| stm32mp131_133_135 TFBGA289 9x9
[IBIS ver]   4.2
[File name]   stm32mp131_133_135_tfbga289.ibs
[File Rev]   3.4
[Date]   06-03-2024
[Source]   Data Created at STMicroelectronics
[Disclaimer]  This information is for modeling purpose only and is
   not guaranteed.
   The information is subject to change without notice.
[Copyright]   Copyright 2024 STMicroelectronics Inc.
|  You might uncomment [Merged Pins] sections if handeled by the simulation tool
[Component] stm32mp131_133_135_tfbga289
[Manufacturer] STMicroelectronics
[Package]
| variable   typ   min   max
R_pkg  0  NA  NA
L_pkg  0  NA  NA
C_pkg  0  NA  NA
[Pin]   signal_name   model_name
H11  BYPASS_REG1V8  nc
G16  DDR_A0  PDDRIO_PAD
L15  DDR_A1  PDDRIO_PAD
J15  DDR_A10  PDDRIO_PAD
L16  DDR_A11  PDDRIO_PAD
L14  DDR_A12  PDDRIO_PAD
E17  DDR_A13  PDDRIO_PAD
L17  DDR_A14  PDDRIO_PAD
K15  DDR_A15  PDDRIO_PAD
G13  DDR_A2  PDDRIO_PAD
G15  DDR_A3  PDDRIO_PAD
P15  DDR_A4  PDDRIO_PAD
F16  DDR_A5  PDDRIO_PAD
M15  DDR_A6  PDDRIO_PAD
F15  DDR_A7  PDDRIO_PAD
M16  DDR_A8  PDDRIO_PAD
F17  DDR_A9  PDDRIO_PAD
N17  DDR_ATO  nc
H15  DDR_BA0  PDDRIO_PAD
M17  DDR_BA1  PDDRIO_PAD
G14  DDR_BA2  PDDRIO_PAD
J17  DDR_CASN  PDDRIO_PAD
L13  DDR_CKE  PDDRIO_PAD
K17  DDR_CLKN  PDDRIO_PAD
K16  DDR_CLKP  PDDRIO_PAD
H16  DDR_CSN  PDDRIO_PAD
A16  DDR_DQ0  PDDRIO_PAD
B15  DDR_DQ1  PDDRIO_PAD
U16  DDR_DQ10  PDDRIO_PAD
R16  DDR_DQ11  PDDRIO_PAD
R15  DDR_DQ12  PDDRIO_PAD
T14  DDR_DQ13  PDDRIO_PAD
T15  DDR_DQ14  PDDRIO_PAD
U15  DDR_DQ15  PDDRIO_PAD
C14  DDR_DQ2  PDDRIO_PAD
C16  DDR_DQ3  PDDRIO_PAD
A15  DDR_DQ4  PDDRIO_PAD
C17  DDR_DQ5  PDDRIO_PAD
D17  DDR_DQ6  PDDRIO_PAD
D16  DDR_DQ7  PDDRIO_PAD
P17  DDR_DQ8  PDDRIO_PAD
R17  DDR_DQ9  PDDRIO_PAD
C15  DDR_DQM0  PDDRIO_PAD
R14  DDR_DQM1  PDDRIO_PAD
B16  DDR_DQS0N  PDIFF_PAD
B17  DDR_DQS0P  PDIFF_PAD
T17  DDR_DQS1N  PDIFF_PAD
T16  DDR_DQS1P  PDIFF_PAD
G17  DDR_ODT  PDDRIO_PAD
J14  DDR_RASN  PDDRIO_PAD
D15  DDR_RESETN  PDDRIO_PAD
J13  DDR_VREF  nc
H17  DDR_WEN  PDDRIO_PAD
P16  DDR_ZQ  nc
R10  NJTRST  io8_ft
K10  NRST  nc
J10  NRST_CORE  nc
L7  PA0  io8_ft
K8  PA1  io8_ft
J12  PA10  io8usb_id_otg20_ft
N5  PA11  io8_ft_i2c
F2  PA12  io8_ft_hslv
K7  PA13  io8_ft
R11  PA14  io8_ft
E7  PA15  io8_ft_hslv
R5  PA2  io8_ft
T7  PA3  io8_ft_hslv
N7  PA4  io8_ft
M7  PA5  io8_ft
R8  PA6  io8_ft_hslv
R6  PA7  io8_ft_hslv
J8  PA8  io8_ft_i2c_hslv
D2  PA9  io8_ft_hslv
M8  PB0  io8_ft
N8  PB1  io8_ft_hslv
G10  PB10  io8_ft_hslv
M6  PB11  io8_ft_hslv_et
A7  PB12  io8_ft_hslv
B10  PB13  io8_ft_i2c_hslv
A12  PB14  io8_ft_hslv
D11  PB15  io8_ft_hslv
K3  PB2  io8_ft_hslv
B11  PB3  io8_ft_hslv
E11  PB4  io8_ft_hslv
F9  PB5  io8_ft_hslv
G3  PB6  io8_ft_hslv
D5  PB7  io8_ft_i2c
G4  PB8  io8_ft_i2c
C10  PB9  io8_ft_i2c_hslv
T4  PC0  io8_ft_hslv
R7  PC1  io8_ft_hslv_et
F11  PC10  io8_ft_i2c_hslv
C12  PC11  io8_ft_i2c_hslv
B13  PC12  io8_ft_hslv
M3  PC13  io8_ft
M1  PC14  io8_ft
M2  PC15  io8_ft
U8  PC2  io8_ft_hslv_et
P7  PC3  io8_ft_hslv
K9  PC4  io8_ft
P8  PC5  io8_ft
A10  PC6  io8_ft_hslv
A9  PC7  io8_ft_hslv
C13  PC8  io8_ft_hslv
G12  PC9  io8_ft_hslv
E1  PD0  io8_ft
C2  PD1  io8_ft_i2c_hslv
D3  PD10  io8_ft_hslv
G1  PD11  io8_ft_hslv
D7  PD12  io8_ft_i2c
N1  PD13  io8_ft_hslv
F7  PD14  io8_ft_i2c_hslv
A5  PD15  io8_ft_hslv
G11  PD2  io8_ft_hslv
G6  PD3  io8_ft_i2c
A2  PD4  io8_ft_hslv
B4  PD5  io8_ft_hslv
G9  PD6  io8_ft
R3  PD7  io8_ft_i2c_hslv
B2  PD8  io8_ft
B5  PD9  io8_ft_hslv
U7  PDR_ON  nc
B3  PE0  io8_ft_hslv
C3  PE1  io8_ft_hslv
C7  PE10  io8_ft
E4  PE11  io8_ft_hslv_et
B1  PE12  io8_ft_hslv
C1  PE13  io8_ft_i2c_hslv
E2  PE14  io8_ft_hslv
A6  PE15  io8_ft_i2c_hslv
T1  PE2  io8_ft_i2c_hslv
B12  PE3  io8_ft_hslv
K1  PE4  io8_ft_hslv
L9  PE5  io8_ft_hslv_et
R2  PE6  io8_ft_hslv_et
C4  PE7  io8_ft_hslv
F8  PE8  io8_ft_i2c
A3  PE9  io8_ft_hslv
A11  PF0  io8_ft_hslv
A8  PF1  io8_ft_i2c_hslv
K2  PF10  io8_ft_hslv
L8  PF11  io8_ft
J9  PF12  io8_ft_hslv_et
T3  PF13  io8_ft
U4  PF14  io8_ft
L10  PF15  io8_ft
B7  PF2  io8_ft_i2c_hslv
B9  PF3  io8_ft_i2c_hslv
P3  PF4  io8_ft_hslv
D1  PF5  io8_ft_hslv
L1  PF6  io8_ft_hslv_et
J7  PF7  io8_ft_hslv_et
H3  PF8  io8_ft_hslv
H9  PF9  io8_ft_hslv
A4  PG0  io8_ft_hslv
P4  PG1  io8_ft_hslv_et
H2  PG10  io8_ft_hslv
R1  PG11  io8_ft_hslv_et
L6  PG12  io8_ft
R9  PG13  io8_ft_hslv_et
T8  PG14  io8_ft_hslv_et
G8  PG15  io8_ft_hslv
U3  PG2  io8_ft
U2  PG3  io8_ft_et_i2c_hslv
C9  PG4  io8_ft_hslv
H1  PG5  io8_ft_hslv
H10  PG6  io8_ft_hslv
C8  PG7  io8_ft_hslv
J3  PG8  io8_ft_hslv
G5  PG9  io8_ft_i2c
P1  PH0  io8_ft
P2  PH1  io8_ft
C11  PH10  io8_ft_hslv
H7  PH11  io8_ft_i2c_hslv
G7  PH12  io8_ft_i2c_hslv
E9  PH13  io8_ft_i2c_hslv
B6  PH14  io8_ft_i2c_hslv
G2  PH2  io8_ft_hslv
T2  PH3  io8_ft_i2c_hslv
T13  PH4  io8_ft
L12  PH5  io8_ft
J6  PH6  io8_ft_i2c_hslv
L3  PH7  io8_ft_i2c_hslv
F1  PH8  io8_ft_i2c_hslv
D9  PH9  io8_ft_hslv
N3  PI0  io8_ft
N4  PI1  io8_ft
J4  PI2  io8_ft
H8  PI3  io8_ft
P11  PI4  io8_ft
N11  PI5  io8_ft
M11  PI6  io8_ft
U13  PI7  io8usb_vbus_otg20_ft
R4  PWR_CPU_ON  io8_ft
U14  PWR_LP  io8_ft
R13  PWR_ON  io8_ft
U12  USB_DM1  nc
U9  USB_DM2  nc
T12  USB_DP1  nc
T9  USB_DP2  nc
M10  USB_RREF  nc
J5  VBAT  power
L4  VDD_ANA  power
C6  VDD  power
F6  VDD_CORE  power
F10  VDD_CORE  power
F12  VDD_CORE  power
H6  VDD_CORE  power
H12  VDD_CORE  power
K12  VDD_CORE  power
M12  VDD_CORE  power
K6  VDD_CORE  power
M9  VDD_CORE  power
D4  VDD_CPU  power
D6  VDD_CPU  power
D8  VDD_CPU  power
E5  VDD_CPU  power
F4  VDD_CPU  power
H4  VDD_CPU  power
D10  VDD  power
D12  VDD  power
D14  VDD_DDR  power
E13  VDD_DDR  power
E15  VDD_DDR  power
F14  VDD_DDR  power
H14  VDD_DDR  power
K14  VDD_DDR  power
M14  VDD_DDR  power
N13  VDD_DDR  power
N15  VDD_DDR  power
P14  VDD_DDR  power
F3  VDD  power
K4  VDD  power
M4  VDD  power
P12  VDD  power
P6  VDD  power
P9  VDD  power
P10  VDD  power
J1  VDD_PLL  power
L11  VDD_PLL2  power
U11  VDD3V3_USBHS  power
U5  VDDA  power
U10  VDDA1V1_REG  power
J11  VDDA1V8_REG  power
A14  VDDSDMMC1  power
A13  VDDSDMMC2  power
T6  VREFN  gnd
U6  VREFP  power
A1  VSS  gnd
A17  VSS  gnd
B8  VSS  gnd
B14  VSS  gnd
C5  VSS  gnd
D13  VSS  gnd
E3  VSS  gnd
E6  VSS  gnd
E8  VSS  gnd
E10  VSS  gnd
E12  VSS  gnd
E14  VSS  gnd
E16  VSS  gnd
F5  VSS  gnd
F13  VSS  gnd
H5  VSS  gnd
H13  VSS  gnd
J16  VSS  gnd
K5  VSS  gnd
K13  VSS  gnd
M5  VSS  gnd
M13  VSS  gnd
N6  VSS  gnd
N9  VSS  gnd
N10  VSS  gnd
N12  VSS  gnd
N14  VSS  gnd
N16  VSS  gnd
P5  VSS  gnd
P13  VSS  gnd
U17  VSS  gnd
L5  VSS_ANA  gnd
L2  VSS  gnd
N2  VSS  gnd
U1  VSS  gnd
J2  VSS_PLL  gnd
K11  VSS_PLL2  gnd
R12  VSS  gnd
T10  VSS  gnd
T11  VSS_USBHS  gnd
T5  VSSA  gnd
[Package Model]   501-bga-9x9-289-210615
[Pin Mapping]   pulldown_ref   pullup_ref   | Comment
H11  nc  nc  | Depending on IO usage
| H11  nc  nc  | Depending on IO usage
G16  gnd  vddddr
L15  gnd  vddddr
J15  gnd  vddddr
L16  gnd  vddddr
L14  gnd  vddddr
E17  gnd  vddddr
L17  gnd  vddddr
K15  gnd  vddddr
G13  gnd  vddddr
G15  gnd  vddddr
P15  gnd  vddddr
F16  gnd  vddddr
M15  gnd  vddddr
F15  gnd  vddddr
M16  gnd  vddddr
F17  gnd  vddddr
N17  nc  nc
H15  gnd  vddddr
M17  gnd  vddddr
G14  gnd  vddddr
J17  gnd  vddddr
L13  gnd  vddddr
K17  gnd  vddddr
K16  gnd  vddddr
H16  gnd  vddddr
A16  gnd  vddddr
B15  gnd  vddddr
U16  gnd  vddddr
R16  gnd  vddddr
R15  gnd  vddddr
T14  gnd  vddddr
T15  gnd  vddddr
U15  gnd  vddddr
C14  gnd  vddddr
C16  gnd  vddddr
A15  gnd  vddddr
C17  gnd  vddddr
D17  gnd  vddddr
D16  gnd  vddddr
P17  gnd  vddddr
R17  gnd  vddddr
C15  gnd  vddddr
R14  gnd  vddddr
B16  gnd  vddddr
B17  gnd  vddddr
T17  gnd  vddddr
T16  gnd  vddddr
G17  gnd  vddddr
J14  gnd  vddddr
D15  gnd  vddddr
J13  nc  nc
H17  gnd  vddddr
P16  nc  nc
R10  gnd  vddio
K10  nc  nc
J10  nc  nc
L7  gnd  vddio
K8  gnd  vddio
J12  gnd  vddio
N5  gnd  vddio
F2  gnd  vddio
K7  gnd  vddio
R11  gnd  vddio
E7  gnd  vddio
R5  gnd  vddio
T7  gnd  vddio
N7  gnd  vddio
M7  gnd  vddio
R8  gnd  vddio
R6  gnd  vddio
J8  gnd  vddio
D2  gnd  vddio
M8  gnd  vddio
N8  gnd  vddio
G10  gnd  vddio
M6  gnd  vddio
A7  gnd  vddio
B10  gnd  vddio
A12  gnd  vdds2  | Depending on IO usage
| A12  gnd  vddio  | Depending on IO usage
D11  gnd  vdds2  | Depending on IO usage
| D11  gnd  vddio  | Depending on IO usage
K3  gnd  vddio
B11  gnd  vdds2  | Depending on IO usage
| B11  gnd  vddio  | Depending on IO usage
E11  gnd  vdds2  | Depending on IO usage
| E11  gnd  vddio  | Depending on IO usage
F9  gnd  vddio
G3  gnd  vddio
D5  gnd  vddio
G4  gnd  vddio
C10  gnd  vddio
T4  gnd  vddio
R7  gnd  vddio
F11  gnd  vdds1  | Depending on IO usage
| F11  gnd  vddio  | Depending on IO usage
C12  gnd  vdds1  | Depending on IO usage
| C12  gnd  vddio  | Depending on IO usage
B13  gnd  vdds1  | Depending on IO usage
| B13  gnd  vddio  | Depending on IO usage
M3  gnd  vddio  | Depending on IO usage
| M3  gnd  vbat  | Depending on IO usage
M1  gnd  vddio  | Depending on IO usage
| M1  gnd  vbat  | Depending on IO usage
M2  gnd  vddio  | Depending on IO usage
| M2  gnd  vbat  | Depending on IO usage
U8  gnd  vddio
P7  gnd  vddio
K9  gnd  vddio
P8  gnd  vddio
A10  gnd  vddio
A9  gnd  vddio
C13  gnd  vdds1  | Depending on IO usage
| C13  gnd  vddio  | Depending on IO usage
G12  gnd  vdds1  | Depending on IO usage
| G12  gnd  vddio  | Depending on IO usage
E1  gnd  vddio
C2  gnd  vddio
D3  gnd  vddio
G1  gnd  vddio
D7  gnd  vddio
N1  gnd  vddio
F7  gnd  vddio
A5  gnd  vddio
G11  gnd  vdds1  | Depending on IO usage
| G11  gnd  vddio  | Depending on IO usage
G6  gnd  vddio
A2  gnd  vddio
B4  gnd  vddio
G9  gnd  vddio
R3  gnd  vddio
B2  gnd  vddio
B5  gnd  vddio
U7  nc  nc
B3  gnd  vddio
C3  gnd  vddio
C7  gnd  vddio
E4  gnd  vddio
B1  gnd  vddio
C1  gnd  vddio
E2  gnd  vddio
A6  gnd  vddio
T1  gnd  vddio
B12  gnd  vdds2  | Depending on IO usage
| B12  gnd  vddio  | Depending on IO usage
K1  gnd  vddio
L9  gnd  vddio
R2  gnd  vddio
C4  gnd  vddio
F8  gnd  vddio
A3  gnd  vddio
A11  gnd  vddio
A8  gnd  vddio
K2  gnd  vddio
L8  gnd  vddio
J9  gnd  vddio
T3  gnd  vddio
U4  gnd  vddio
L10  gnd  vddio
B7  gnd  vddio
B9  gnd  vddio
P3  gnd  vddio
D1  gnd  vddio
L1  gnd  vddio
J7  gnd  vddio
H3  gnd  vddio
H9  gnd  vddio
A4  gnd  vddio
P4  gnd  vddio
H2  gnd  vddio
R1  gnd  vddio
L6  gnd  vddio
R9  gnd  vddio
T8  gnd  vddio
G8  gnd  vddio
U3  gnd  vddio
U2  gnd  vddio
C9  gnd  vddio
H1  gnd  vddio
H10  gnd  vdds2  | Depending on IO usage
| H10  gnd  vddio  | Depending on IO usage
C8  gnd  vddio
J3  gnd  vddio
G5  gnd  vddio
P1  gnd  vddio
P2  gnd  vddio
C11  gnd  vddio
H7  gnd  vddio
G7  gnd  vddio
E9  gnd  vddio
B6  gnd  vddio
G2  gnd  vddio
T2  gnd  vddio
T13  gnd  vddio
L12  gnd  vddio
J6  gnd  vddio
L3  gnd  vddio
F1  gnd  vddio
D9  gnd  vddio
N3  gnd  vddio
N4  gnd  vddio  | Depending on IO usage
| N4  gnd  vbat  | Depending on IO usage
J4  gnd  vddio  | Depending on IO usage
| J4  gnd  vbat  | Depending on IO usage
H8  gnd  vddio  | Depending on IO usage
| H8  gnd  vbat  | Depending on IO usage
P11  gnd  vddio
N11  gnd  vddio
M11  gnd  vddio
U13  gnd  vddio
R4  gnd  vddio
U14  gnd  vddio
R13  gnd  vddio
U12  nc  nc  | Depending on IO usage
| U12  nc  nc  | Depending on IO usage
U9  nc  nc  | Depending on IO usage
| U9  nc  nc  | Depending on IO usage
T12  nc  nc  | Depending on IO usage
| T12  nc  nc  | Depending on IO usage
T9  nc  nc  | Depending on IO usage
| T9  nc  nc  | Depending on IO usage
M10  nc  nc  | Depending on IO usage
| M10  nc  nc  | Depending on IO usage
J5  nc  vbat
L4  nc  vddana
C6  nc  vddio
F6  nc  vddio  | Depending on IO usage
| F6  nc  vbat  | Depending on IO usage
F10  nc  vddio  | Depending on IO usage
| F10  nc  vbat  | Depending on IO usage
F12  nc  vddio  | Depending on IO usage
| F12  nc  vbat  | Depending on IO usage
H6  nc  vddio  | Depending on IO usage
| H6  nc  vbat  | Depending on IO usage
H12  nc  vddio  | Depending on IO usage
| H12  nc  vbat  | Depending on IO usage
K12  nc  vddio  | Depending on IO usage
| K12  nc  vbat  | Depending on IO usage
M12  nc  vddio  | Depending on IO usage
| M12  nc  vbat  | Depending on IO usage
K6  nc  vddio  | Depending on IO usage
| K6  nc  vbat  | Depending on IO usage
M9  nc  vddio  | Depending on IO usage
| M9  nc  vbat  | Depending on IO usage
D4  nc  vddcpu
D6  nc  vddcpu
D8  nc  vddcpu
E5  nc  vddcpu
F4  nc  vddcpu
H4  nc  vddcpu
D10  nc  vddio
D12  nc  vddio
D14  nc  vddddr
E13  nc  vddddr
E15  nc  vddddr
F14  nc  vddddr
H14  nc  vddddr
K14  nc  vddddr
M14  nc  vddddr
N13  nc  vddddr
N15  nc  vddddr
P14  nc  vddddr
F3  nc  vddio
K4  nc  vddio
M4  nc  vddio
P12  nc  vddio
P6  nc  vddio
P9  nc  vddio
P10  nc  vddio
J1  nc  vddpll
L11  nc  vddpll2
U11  nc  vdd3v3usbhs
U5  nc  vdda
U10  nc  vdda1v1
J11  nc  vdda1v8
A14  nc  vdds1
A13  nc  vdds2
T6  gnd  nc
U6  nc  vddio
A1  gnd  nc
A17  gnd  nc
B8  gnd  nc
B14  gnd  nc
C5  gnd  nc
D13  gnd  nc
E3  gnd  nc
E6  gnd  nc
E8  gnd  nc
E10  gnd  nc
E12  gnd  nc
E14  gnd  nc
E16  gnd  nc
F5  gnd  nc
F13  gnd  nc
H5  gnd  nc
H13  gnd  nc
J16  gnd  nc
K5  gnd  nc
K13  gnd  nc
M5  gnd  nc
M13  gnd  nc
N6  gnd  nc
N9  gnd  nc
N10  gnd  nc
N12  gnd  nc
N14  gnd  nc
N16  gnd  nc
P5  gnd  nc
P13  gnd  nc
U17  gnd  nc
L5  gnd  nc
L2  gnd  nc
N2  gnd  nc
U1  gnd  nc
J2  gnd  nc
K11  gnd  nc
R12  gnd  nc
T10  gnd  nc
T11  gnd  nc
T5  gnd  nc
[Diff_pin]   inv_pin   vdiff   tdelay_typ   tdelay_min   tdelay_max
   K16   K17   0.320V   0ns   NA   NA   |CK
   B17   B16   0.320V   0ns   NA   NA   |DQS0
   T16   T17   0.320V   0ns   NA   NA   |DQS1
[Model Selector] PDIFF_PAD
MSD_D3RF2_18   DDR2 MSD_D3R_PDIFF Z0=18-Ohm
MSD_D3RF2_40   DDR2 MSD_D3R_PDIFF Z0=40-Ohm
MSD_D3RF2_48   DDR2 MSD_D3R_PDIFF Z0=48-Ohm
MSD_D3RF2_ODT150   DDR2 MSD_D3R_PDIFF cell 150-Ohm ODT Receiver
MSD_D3RF2_ODT50   DDR2 MSD_D3R_PDIFF cell 50-Ohm ODT Receiver
MSD_D3RF2_ODT75   DDR2 MSD_D3R_PDIFF cell 75-Ohm ODT Receiver
MSD_D3RF2_ODTOFF   DDR2 MSD_D3R_PDIFF cell ODT off Receiver
MSD_D3RF3_34   DDR3 MSD_D3R_PDIFF cell  Z0=34-Ohm
MSD_D3RF3_40   DDR3 MSD_D3R_PDIFF cell  Z0=40-Ohm
MSD_D3RF3_48   DDR3 MSD_D3R_PDIFF cell  Z0=48-Ohm
MSD_D3RF3L_34   DDR3L MSD_D3R_PDIFF cell  Z0=34-Ohm
MSD_D3RF3L_40   DDR3L MSD_D3R_PDIFF cell  Z0=40-Ohm
MSD_D3RF3L_48   DDR3L MSD_D3R_PDIFF cell  Z0=48-Ohm
MSD_D3RF3L_ODT120   DDR3L MSD_D3R_PDIFF cell 120-Ohm ODT Receiver
MSD_D3RF3L_ODT40   DDR3L MSD_D3R_PDIFF cell 40-Ohm ODT Receiver
MSD_D3RF3L_ODT60   DDR3L MSD_D3R_PDIFF cell 60-Ohm ODT Receiver
MSD_D3RF3L_ODTOFF   DDR3L MSD_D3R_PDIFF cell ODT off Receiver
MSD_D3RF3_ODT120   DDR3 MSD_D3R_PDIFF cell 120-Ohm ODT Receiver
MSD_D3RF3_ODT40   DDR3 MSD_D3R_PDIFF cell 40-Ohm ODT Receiver
MSD_D3RF3_ODT60   DDR3 MSD_D3R_PDIFF cell 60-Ohm ODT Receiver
MSD_D3RF3_ODTOFF   DDR3 MSD_D3R_PDIFF cell ODT off Receiver
MSD_D3RFL2_34   LPDDR2 MSD_D3R_PDIFF cell  Z0=34-Ohm
MSD_D3RFL2_40   LPDDR2 MSD_D3R_PDIFF cell  Z0=40-Ohm
MSD_D3RFL2_48   LPDDR2 MSD_D3R_PDIFF cell  Z0=48-Ohm
MSD_D3RFL2_60   LPDDR2 MSD_D3R_PDIFF cell  Z0=60-Ohm
MSD_D3RFL2_80   LPDDR2 MSD_D3R_PDIFF cell  Z0=80-Ohm
MSD_D3RFL2_ODTOFF   LPDDR2 MSD_D3R_PDIFF cell ODT off Receiver
MSD_D3RFL_48   LPDDR MSD_D3R_PDIFF cell  Z0=48-Ohm
MSD_D3RFL_ODTOFF   LPDDR MSD_D3R_PDIFF cell ODT off Receiver
MSD_D3RF2_18_OPEN   DDR2 MSD_D3R_PDIFF_PDQSR Z0=18-Ohm
MSD_D3RF2_40_OPEN   DDR2 MSD_D3R_PDIFF_PDQSR Z0=40-Ohm
MSD_D3RF2_48_OPEN   DDR2 MSD_D3R_PDIFF_PDQSR Z0=48-Ohm
MSD_D3RF2_18_PD344   DDR2 MSD_D3R_PDIFF_PDQSR Z0=18-Ohm
MSD_D3RF2_40_PD344   DDR2 MSD_D3R_PDIFF_PDQSR Z0=40-Ohm
MSD_D3RF2_48_PD344   DDR2 MSD_D3R_PDIFF_PDQSR Z0=48-Ohm
MSD_D3RF2_18_PD393   DDR2 MSD_D3R_PDIFF_PDQSR Z0=18-Ohm
MSD_D3RF2_40_PD393   DDR2 MSD_D3R_PDIFF_PDQSR Z0=40-Ohm
MSD_D3RF2_48_PD393   DDR2 MSD_D3R_PDIFF_PDQSR Z0=48-Ohm
MSD_D3RF2_18_PD458   DDR2 MSD_D3R_PDIFF_PDQSR Z0=18-Ohm
MSD_D3RF2_40_PD458   DDR2 MSD_D3R_PDIFF_PDQSR Z0=40-Ohm
MSD_D3RF2_48_PD458   DDR2 MSD_D3R_PDIFF_PDQSR Z0=48-Ohm
MSD_D3RF2_18_PD500   DDR2 MSD_D3R_PDIFF_PDQSR Z0=18-Ohm
MSD_D3RF2_40_PD500   DDR2 MSD_D3R_PDIFF_PDQSR Z0=40-Ohm
MSD_D3RF2_48_PD500   DDR2 MSD_D3R_PDIFF_PDQSR Z0=48-Ohm
MSD_D3RF2_18_PD550   DDR2 MSD_D3R_PDIFF_PDQSR Z0=18-Ohm
MSD_D3RF2_40_PD550   DDR2 MSD_D3R_PDIFF_PDQSR Z0=40-Ohm
MSD_D3RF2_48_PD550   DDR2 MSD_D3R_PDIFF_PDQSR Z0=48-Ohm
MSD_D3RF2_18_PD611   DDR2 MSD_D3R_PDIFF_PDQSR Z0=18-Ohm
MSD_D3RF2_40_PD611   DDR2 MSD_D3R_PDIFF_PDQSR Z0=40-Ohm
MSD_D3RF2_48_PD611   DDR2 MSD_D3R_PDIFF_PDQSR Z0=48-Ohm
MSD_D3RF2_18_PD688   DDR2 MSD_D3R_PDIFF_PDQSR Z0=18-Ohm
MSD_D3RF2_40_PD688   DDR2 MSD_D3R_PDIFF_PDQSR Z0=40-Ohm
MSD_D3RF2_48_PD688   DDR2 MSD_D3R_PDIFF_PDQSR Z0=48-Ohm
MSD_D3RF2_18_PU344   DDR2 MSD_D3R_PDIFF_PDQSR Z0=18-Ohm
MSD_D3RF2_40_PU344   DDR2 MSD_D3R_PDIFF_PDQSR Z0=40-Ohm
MSD_D3RF2_48_PU344   DDR2 MSD_D3R_PDIFF_PDQSR Z0=48-Ohm
MSD_D3RF2_18_PU393   DDR2 MSD_D3R_PDIFF_PDQSR Z0=18-Ohm
MSD_D3RF2_40_PU393   DDR2 MSD_D3R_PDIFF_PDQSR Z0=40-Ohm
MSD_D3RF2_48_PU393   DDR2 MSD_D3R_PDIFF_PDQSR Z0=48-Ohm
MSD_D3RF2_18_PU458   DDR2 MSD_D3R_PDIFF_PDQSR Z0=18-Ohm
MSD_D3RF2_40_PU458   DDR2 MSD_D3R_PDIFF_PDQSR Z0=40-Ohm
MSD_D3RF2_48_PU458   DDR2 MSD_D3R_PDIFF_PDQSR Z0=48-Ohm
MSD_D3RF2_18_PU500   DDR2 MSD_D3R_PDIFF_PDQSR Z0=18-Ohm
MSD_D3RF2_40_PU500   DDR2 MSD_D3R_PDIFF_PDQSR Z0=40-Ohm
MSD_D3RF2_48_PU500   DDR2 MSD_D3R_PDIFF_PDQSR Z0=48-Ohm
MSD_D3RF2_18_PU550   DDR2 MSD_D3R_PDIFF_PDQSR Z0=18-Ohm
MSD_D3RF2_40_PU550   DDR2 MSD_D3R_PDIFF_PDQSR Z0=40-Ohm
MSD_D3RF2_48_PU550   DDR2 MSD_D3R_PDIFF_PDQSR Z0=48-Ohm
MSD_D3RF2_18_PU611   DDR2 MSD_D3R_PDIFF_PDQSR Z0=18-Ohm
MSD_D3RF2_40_PU611   DDR2 MSD_D3R_PDIFF_PDQSR Z0=40-Ohm
MSD_D3RF2_48_PU611   DDR2 MSD_D3R_PDIFF_PDQSR Z0=48-Ohm
MSD_D3RF2_18_PU688   DDR2 MSD_D3R_PDIFF_PDQSR Z0=18-Ohm
MSD_D3RF2_40_PU688   DDR2 MSD_D3R_PDIFF_PDQSR Z0=40-Ohm
MSD_D3RF2_48_PU688   DDR2 MSD_D3R_PDIFF_PDQSR Z0=48-Ohm
MSD_D3RF2_18_PWRDWN   DDR2 MSD_D3R_PDIFF_PDQSR Z0=18-Ohm
MSD_D3RF2_40_PWRDWN   DDR2 MSD_D3R_PDIFF_PDQSR Z0=40-Ohm
MSD_D3RF2_48_PWRDWN   DDR2 MSD_D3R_PDIFF_PDQSR Z0=48-Ohm
MSD_D3RF3_34_OPEN   DDR3 MSD_D3R_PDIFF_PDQSR cell  Z0=34-Ohm
MSD_D3RF3_40_OPEN   DDR3 MSD_D3R_PDIFF_PDQSR cell  Z0=40-Ohm
MSD_D3RF3_48_OPEN   DDR3 MSD_D3R_PDIFF_PDQSR cell  Z0=48-Ohm
MSD_D3RF3_34_PD344   DDR3 MSD_D3R_PDIFF_PDQSR cell  Z0=34-Ohm
MSD_D3RF3_40_PD344   DDR3 MSD_D3R_PDIFF_PDQSR cell  Z0=40-Ohm
MSD_D3RF3_48_PD344   DDR3 MSD_D3R_PDIFF_PDQSR cell  Z0=48-Ohm
MSD_D3RF3_34_PD393   DDR3 MSD_D3R_PDIFF_PDQSR cell  Z0=34-Ohm
MSD_D3RF3_40_PD393   DDR3 MSD_D3R_PDIFF_PDQSR cell  Z0=40-Ohm
MSD_D3RF3_48_PD393   DDR3 MSD_D3R_PDIFF_PDQSR cell  Z0=48-Ohm
MSD_D3RF3_34_PD458   DDR3 MSD_D3R_PDIFF_PDQSR cell  Z0=34-Ohm
MSD_D3RF3_40_PD458   DDR3 MSD_D3R_PDIFF_PDQSR cell  Z0=40-Ohm
MSD_D3RF3_48_PD458   DDR3 MSD_D3R_PDIFF_PDQSR cell  Z0=48-Ohm
MSD_D3RF3_34_PD500   DDR3 MSD_D3R_PDIFF_PDQSR cell  Z0=34-Ohm
MSD_D3RF3_40_PD500   DDR3 MSD_D3R_PDIFF_PDQSR cell  Z0=40-Ohm
MSD_D3RF3_48_PD500   DDR3 MSD_D3R_PDIFF_PDQSR cell  Z0=48-Ohm
MSD_D3RF3_34_PD550   DDR3 MSD_D3R_PDIFF_PDQSR cell  Z0=34-Ohm
MSD_D3RF3_40_PD550   DDR3 MSD_D3R_PDIFF_PDQSR cell  Z0=40-Ohm
MSD_D3RF3_48_PD550   DDR3 MSD_D3R_PDIFF_PDQSR cell  Z0=48-Ohm
MSD_D3RF3_34_PD611   DDR3 MSD_D3R_PDIFF_PDQSR cell  Z0=34-Ohm
MSD_D3RF3_40_PD611   DDR3 MSD_D3R_PDIFF_PDQSR cell  Z0=40-Ohm
MSD_D3RF3_48_PD611   DDR3 MSD_D3R_PDIFF_PDQSR cell  Z0=48-Ohm
MSD_D3RF3_34_PD688   DDR3 MSD_D3R_PDIFF_PDQSR cell  Z0=34-Ohm
MSD_D3RF3_40_PD688   DDR3 MSD_D3R_PDIFF_PDQSR cell  Z0=40-Ohm
MSD_D3RF3_48_PD688   DDR3 MSD_D3R_PDIFF_PDQSR cell  Z0=48-Ohm
MSD_D3RF3_34_PU344   DDR3 MSD_D3R_PDIFF_PDQSR cell  Z0=34-Ohm
MSD_D3RF3_40_PU344   DDR3 MSD_D3R_PDIFF_PDQSR cell  Z0=40-Ohm
MSD_D3RF3_48_PU344   DDR3 MSD_D3R_PDIFF_PDQSR cell  Z0=48-Ohm
MSD_D3RF3_34_PU393   DDR3 MSD_D3R_PDIFF_PDQSR cell  Z0=34-Ohm
MSD_D3RF3_40_PU393   DDR3 MSD_D3R_PDIFF_PDQSR cell  Z0=40-Ohm
MSD_D3RF3_48_PU393   DDR3 MSD_D3R_PDIFF_PDQSR cell  Z0=48-Ohm
MSD_D3RF3_34_PU458   DDR3 MSD_D3R_PDIFF_PDQSR cell  Z0=34-Ohm
MSD_D3RF3_40_PU458   DDR3 MSD_D3R_PDIFF_PDQSR cell  Z0=40-Ohm
MSD_D3RF3_48_PU458   DDR3 MSD_D3R_PDIFF_PDQSR cell  Z0=48-Ohm
MSD_D3RF3_34_PU500   DDR3 MSD_D3R_PDIFF_PDQSR cell  Z0=34-Ohm
MSD_D3RF3_40_PU500   DDR3 MSD_D3R_PDIFF_PDQSR cell  Z0=40-Ohm
MSD_D3RF3_48_PU500   DDR3 MSD_D3R_PDIFF_PDQSR cell  Z0=48-Ohm
MSD_D3RF3_34_PU550   DDR3 MSD_D3R_PDIFF_PDQSR cell  Z0=34-Ohm
MSD_D3RF3_40_PU550   DDR3 MSD_D3R_PDIFF_PDQSR cell  Z0=40-Ohm
MSD_D3RF3_48_PU550   DDR3 MSD_D3R_PDIFF_PDQSR cell  Z0=48-Ohm
MSD_D3RF3_34_PU611   DDR3 MSD_D3R_PDIFF_PDQSR cell  Z0=34-Ohm
MSD_D3RF3_40_PU611   DDR3 MSD_D3R_PDIFF_PDQSR cell  Z0=40-Ohm
MSD_D3RF3_48_PU611   DDR3 MSD_D3R_PDIFF_PDQSR cell  Z0=48-Ohm
MSD_D3RF3_34_PU688   DDR3 MSD_D3R_PDIFF_PDQSR cell  Z0=34-Ohm
MSD_D3RF3_40_PU688   DDR3 MSD_D3R_PDIFF_PDQSR cell  Z0=40-Ohm
MSD_D3RF3_48_PU688   DDR3 MSD_D3R_PDIFF_PDQSR cell  Z0=48-Ohm
MSD_D3RF3_34_PWRDWN   DDR3 MSD_D3R_PDIFF_PDQSR cell  Z0=34-Ohm
MSD_D3RF3_40_PWRDWN   DDR3 MSD_D3R_PDIFF_PDQSR cell  Z0=40-Ohm
MSD_D3RF3_48_PWRDWN   DDR3 MSD_D3R_PDIFF_PDQSR cell  Z0=48-Ohm
MSD_D3RF3L_34_OPEN   DDR3L MSD_D3R_PDIFF_PDQSR cell  Z0=34-Ohm
MSD_D3RF3L_40_OPEN   DDR3L MSD_D3R_PDIFF_PDQSR cell  Z0=40-Ohm
MSD_D3RF3L_48_OPEN   DDR3L MSD_D3R_PDIFF_PDQSR cell  Z0=48-Ohm
MSD_D3RF3L_34_PD344   DDR3L MSD_D3R_PDIFF_PDQSR cell  Z0=34-Ohm
MSD_D3RF3L_40_PD344   DDR3L MSD_D3R_PDIFF_PDQSR cell  Z0=40-Ohm
MSD_D3RF3L_48_PD344   DDR3L MSD_D3R_PDIFF_PDQSR cell  Z0=48-Ohm
MSD_D3RF3L_34_PD393   DDR3L MSD_D3R_PDIFF_PDQSR cell  Z0=34-Ohm
MSD_D3RF3L_40_PD393   DDR3L MSD_D3R_PDIFF_PDQSR cell  Z0=40-Ohm
MSD_D3RF3L_48_PD393   DDR3L MSD_D3R_PDIFF_PDQSR cell  Z0=48-Ohm
MSD_D3RF3L_34_PD458   DDR3L MSD_D3R_PDIFF_PDQSR cell  Z0=34-Ohm
MSD_D3RF3L_40_PD458   DDR3L MSD_D3R_PDIFF_PDQSR cell  Z0=40-Ohm
MSD_D3RF3L_48_PD458   DDR3L MSD_D3R_PDIFF_PDQSR cell  Z0=48-Ohm
MSD_D3RF3L_34_PD500   DDR3L MSD_D3R_PDIFF_PDQSR cell  Z0=34-Ohm
MSD_D3RF3L_40_PD500   DDR3L MSD_D3R_PDIFF_PDQSR cell  Z0=40-Ohm
MSD_D3RF3L_48_PD500   DDR3L MSD_D3R_PDIFF_PDQSR cell  Z0=48-Ohm
MSD_D3RF3L_34_PD550   DDR3L MSD_D3R_PDIFF_PDQSR cell  Z0=34-Ohm
MSD_D3RF3L_40_PD550   DDR3L MSD_D3R_PDIFF_PDQSR cell  Z0=40-Ohm
MSD_D3RF3L_48_PD550   DDR3L MSD_D3R_PDIFF_PDQSR cell  Z0=48-Ohm
MSD_D3RF3L_34_PD611   DDR3L MSD_D3R_PDIFF_PDQSR cell  Z0=34-Ohm
MSD_D3RF3L_40_PD611   DDR3L MSD_D3R_PDIFF_PDQSR cell  Z0=40-Ohm
MSD_D3RF3L_48_PD611   DDR3L MSD_D3R_PDIFF_PDQSR cell  Z0=48-Ohm
MSD_D3RF3L_34_PD688   DDR3L MSD_D3R_PDIFF_PDQSR cell  Z0=34-Ohm
MSD_D3RF3L_40_PD688   DDR3L MSD_D3R_PDIFF_PDQSR cell  Z0=40-Ohm
MSD_D3RF3L_48_PD688   DDR3L MSD_D3R_PDIFF_PDQSR cell  Z0=48-Ohm
MSD_D3RF3L_34_PU344   DDR3L MSD_D3R_PDIFF_PDQSR cell  Z0=34-Ohm
MSD_D3RF3L_40_PU344   DDR3L MSD_D3R_PDIFF_PDQSR cell  Z0=40-Ohm
MSD_D3RF3L_48_PU344   DDR3L MSD_D3R_PDIFF_PDQSR cell  Z0=48-Ohm
MSD_D3RF3L_34_PU393   DDR3L MSD_D3R_PDIFF_PDQSR cell  Z0=34-Ohm
MSD_D3RF3L_40_PU393   DDR3L MSD_D3R_PDIFF_PDQSR cell  Z0=40-Ohm
MSD_D3RF3L_48_PU393   DDR3L MSD_D3R_PDIFF_PDQSR cell  Z0=48-Ohm
MSD_D3RF3L_34_PU458   DDR3L MSD_D3R_PDIFF_PDQSR cell  Z0=34-Ohm
MSD_D3RF3L_40_PU458   DDR3L MSD_D3R_PDIFF_PDQSR cell  Z0=40-Ohm
MSD_D3RF3L_48_PU458   DDR3L MSD_D3R_PDIFF_PDQSR cell  Z0=48-Ohm
MSD_D3RF3L_34_PU500   DDR3L MSD_D3R_PDIFF_PDQSR cell  Z0=34-Ohm
MSD_D3RF3L_40_PU500   DDR3L MSD_D3R_PDIFF_PDQSR cell  Z0=40-Ohm
MSD_D3RF3L_48_PU500   DDR3L MSD_D3R_PDIFF_PDQSR cell  Z0=48-Ohm
MSD_D3RF3L_34_PU550   DDR3L MSD_D3R_PDIFF_PDQSR cell  Z0=34-Ohm
MSD_D3RF3L_40_PU550   DDR3L MSD_D3R_PDIFF_PDQSR cell  Z0=40-Ohm
MSD_D3RF3L_48_PU550   DDR3L MSD_D3R_PDIFF_PDQSR cell  Z0=48-Ohm
MSD_D3RF3L_34_PU611   DDR3L MSD_D3R_PDIFF_PDQSR cell  Z0=34-Ohm
MSD_D3RF3L_40_PU611   DDR3L MSD_D3R_PDIFF_PDQSR cell  Z0=40-Ohm
MSD_D3RF3L_48_PU611   DDR3L MSD_D3R_PDIFF_PDQSR cell  Z0=48-Ohm
MSD_D3RF3L_34_PU688   DDR3L MSD_D3R_PDIFF_PDQSR cell  Z0=34-Ohm
MSD_D3RF3L_40_PU688   DDR3L MSD_D3R_PDIFF_PDQSR cell  Z0=40-Ohm
MSD_D3RF3L_48_PU688   DDR3L MSD_D3R_PDIFF_PDQSR cell  Z0=48-Ohm
MSD_D3RF3L_34_PWRDWN   DDR3L MSD_D3R_PDIFF_PDQSR cell  Z0=34-Ohm
MSD_D3RF3L_40_PWRDWN   DDR3L MSD_D3R_PDIFF_PDQSR cell  Z0=40-Ohm
MSD_D3RF3L_48_PWRDWN   DDR3L MSD_D3R_PDIFF_PDQSR cell  Z0=48-Ohm
MSD_D3RFL2_34_OPEN   LPDDR2 MSD_D3R_PDIFF_PDQSR cell  Z0=34-Ohm
MSD_D3RFL2_40_OPEN   LPDDR2 MSD_D3R_PDIFF_PDQSR cell  Z0=40-Ohm
MSD_D3RFL2_48_OPEN   LPDDR2 MSD_D3R_PDIFF_PDQSR cell  Z0=48-Ohm
MSD_D3RFL2_60_OPEN   LPDDR2 MSD_D3R_PDIFF_PDQSR cell  Z0=60-Ohm
MSD_D3RFL2_80_OPEN   LPDDR2 MSD_D3R_PDIFF_PDQSR cell  Z0=80-Ohm
MSD_D3RFL_48_OPEN   LPDDR MSD_D3R_PDIFF_PDQSR cell  Z0=48-Ohm
MSD_D3RFL2_34_PD344   LPDDR2 MSD_D3R_PDIFF_PDQSR cell  Z0=34-Ohm
MSD_D3RFL2_40_PD344   LPDDR2 MSD_D3R_PDIFF_PDQSR cell  Z0=40-Ohm
MSD_D3RFL2_48_PD344   LPDDR2 MSD_D3R_PDIFF_PDQSR cell  Z0=48-Ohm
MSD_D3RFL2_60_PD344   LPDDR2 MSD_D3R_PDIFF_PDQSR cell  Z0=60-Ohm
MSD_D3RFL2_80_PD344   LPDDR2 MSD_D3R_PDIFF_PDQSR cell  Z0=80-Ohm
MSD_D3RFL_48_PD344   LPDDR MSD_D3R_PDIFF_PDQSR cell  Z0=48-Ohm
MSD_D3RFL2_34_PD393   LPDDR2 MSD_D3R_PDIFF_PDQSR cell  Z0=34-Ohm
MSD_D3RFL2_40_PD393   LPDDR2 MSD_D3R_PDIFF_PDQSR cell  Z0=40-Ohm
MSD_D3RFL2_48_PD393   LPDDR2 MSD_D3R_PDIFF_PDQSR cell  Z0=48-Ohm
MSD_D3RFL2_60_PD393   LPDDR2 MSD_D3R_PDIFF_PDQSR cell  Z0=60-Ohm
MSD_D3RFL2_80_PD393   LPDDR2 MSD_D3R_PDIFF_PDQSR cell  Z0=80-Ohm
MSD_D3RFL_48_PD393   LPDDR MSD_D3R_PDIFF_PDQSR cell  Z0=48-Ohm
MSD_D3RFL2_34_PD458   LPDDR2 MSD_D3R_PDIFF_PDQSR cell  Z0=34-Ohm
MSD_D3RFL2_40_PD458   LPDDR2 MSD_D3R_PDIFF_PDQSR cell  Z0=40-Ohm
MSD_D3RFL2_48_PD458   LPDDR2 MSD_D3R_PDIFF_PDQSR cell  Z0=48-Ohm
MSD_D3RFL2_60_PD458   LPDDR2 MSD_D3R_PDIFF_PDQSR cell  Z0=60-Ohm
MSD_D3RFL2_80_PD458   LPDDR2 MSD_D3R_PDIFF_PDQSR cell  Z0=80-Ohm
MSD_D3RFL_48_PD458   LPDDR MSD_D3R_PDIFF_PDQSR cell  Z0=48-Ohm
MSD_D3RFL2_34_PD500   LPDDR2 MSD_D3R_PDIFF_PDQSR cell  Z0=34-Ohm
MSD_D3RFL2_40_PD500   LPDDR2 MSD_D3R_PDIFF_PDQSR cell  Z0=40-Ohm
MSD_D3RFL2_48_PD500   LPDDR2 MSD_D3R_PDIFF_PDQSR cell  Z0=48-Ohm
MSD_D3RFL2_60_PD500   LPDDR2 MSD_D3R_PDIFF_PDQSR cell  Z0=60-Ohm
MSD_D3RFL2_80_PD500   LPDDR2 MSD_D3R_PDIFF_PDQSR cell  Z0=80-Ohm
MSD_D3RFL_48_PD500   LPDDR MSD_D3R_PDIFF_PDQSR cell  Z0=48-Ohm
MSD_D3RFL2_34_PD550   LPDDR2 MSD_D3R_PDIFF_PDQSR cell  Z0=34-Ohm
MSD_D3RFL2_40_PD550   LPDDR2 MSD_D3R_PDIFF_PDQSR cell  Z0=40-Ohm
MSD_D3RFL2_48_PD550   LPDDR2 MSD_D3R_PDIFF_PDQSR cell  Z0=48-Ohm
MSD_D3RFL2_60_PD550   LPDDR2 MSD_D3R_PDIFF_PDQSR cell  Z0=60-Ohm
MSD_D3RFL2_80_PD550   LPDDR2 MSD_D3R_PDIFF_PDQSR cell  Z0=80-Ohm
MSD_D3RFL_48_PD550   LPDDR MSD_D3R_PDIFF_PDQSR cell  Z0=48-Ohm
MSD_D3RFL2_34_PD611   LPDDR2 MSD_D3R_PDIFF_PDQSR cell  Z0=34-Ohm
MSD_D3RFL2_40_PD611   LPDDR2 MSD_D3R_PDIFF_PDQSR cell  Z0=40-Ohm
MSD_D3RFL2_48_PD611   LPDDR2 MSD_D3R_PDIFF_PDQSR cell  Z0=48-Ohm
MSD_D3RFL2_60_PD611   LPDDR2 MSD_D3R_PDIFF_PDQSR cell  Z0=60-Ohm
MSD_D3RFL2_80_PD611   LPDDR2 MSD_D3R_PDIFF_PDQSR cell  Z0=80-Ohm
MSD_D3RFL_48_PD611   LPDDR MSD_D3R_PDIFF_PDQSR cell  Z0=48-Ohm
MSD_D3RFL2_34_PD688   LPDDR2 MSD_D3R_PDIFF_PDQSR cell  Z0=34-Ohm
MSD_D3RFL2_40_PD688   LPDDR2 MSD_D3R_PDIFF_PDQSR cell  Z0=40-Ohm
MSD_D3RFL2_48_PD688   LPDDR2 MSD_D3R_PDIFF_PDQSR cell  Z0=48-Ohm
MSD_D3RFL2_60_PD688   LPDDR2 MSD_D3R_PDIFF_PDQSR cell  Z0=60-Ohm
MSD_D3RFL2_80_PD688   LPDDR2 MSD_D3R_PDIFF_PDQSR cell  Z0=80-Ohm
MSD_D3RFL_48_PD688   LPDDR MSD_D3R_PDIFF_PDQSR cell  Z0=48-Ohm
MSD_D3RFL2_34_PU344   LPDDR2 MSD_D3R_PDIFF_PDQSR cell  Z0=34-Ohm
MSD_D3RFL2_40_PU344   LPDDR2 MSD_D3R_PDIFF_PDQSR cell  Z0=40-Ohm
MSD_D3RFL2_48_PU344   LPDDR2 MSD_D3R_PDIFF_PDQSR cell  Z0=48-Ohm
MSD_D3RFL2_60_PU344   LPDDR2 MSD_D3R_PDIFF_PDQSR cell  Z0=60-Ohm
MSD_D3RFL2_80_PU344   LPDDR2 MSD_D3R_PDIFF_PDQSR cell  Z0=80-Ohm
MSD_D3RFL_48_PU344   LPDDR MSD_D3R_PDIFF_PDQSR cell  Z0=48-Ohm
MSD_D3RFL2_34_PU393   LPDDR2 MSD_D3R_PDIFF_PDQSR cell  Z0=34-Ohm
MSD_D3RFL2_40_PU393   LPDDR2 MSD_D3R_PDIFF_PDQSR cell  Z0=40-Ohm
MSD_D3RFL2_48_PU393   LPDDR2 MSD_D3R_PDIFF_PDQSR cell  Z0=48-Ohm
MSD_D3RFL2_60_PU393   LPDDR2 MSD_D3R_PDIFF_PDQSR cell  Z0=60-Ohm
MSD_D3RFL2_80_PU393   LPDDR2 MSD_D3R_PDIFF_PDQSR cell  Z0=80-Ohm
MSD_D3RFL_48_PU393   LPDDR MSD_D3R_PDIFF_PDQSR cell  Z0=48-Ohm
MSD_D3RFL2_34_PU458   LPDDR2 MSD_D3R_PDIFF_PDQSR cell  Z0=34-Ohm
MSD_D3RFL2_40_PU458   LPDDR2 MSD_D3R_PDIFF_PDQSR cell  Z0=40-Ohm
MSD_D3RFL2_48_PU458   LPDDR2 MSD_D3R_PDIFF_PDQSR cell  Z0=48-Ohm
MSD_D3RFL2_60_PU458   LPDDR2 MSD_D3R_PDIFF_PDQSR cell  Z0=60-Ohm
MSD_D3RFL2_80_PU458   LPDDR2 MSD_D3R_PDIFF_PDQSR cell  Z0=80-Ohm
MSD_D3RFL_48_PU458   LPDDR MSD_D3R_PDIFF_PDQSR cell  Z0=48-Ohm
MSD_D3RFL2_34_PU500   LPDDR2 MSD_D3R_PDIFF_PDQSR cell  Z0=34-Ohm
MSD_D3RFL2_40_PU500   LPDDR2 MSD_D3R_PDIFF_PDQSR cell  Z0=40-Ohm
MSD_D3RFL2_48_PU500   LPDDR2 MSD_D3R_PDIFF_PDQSR cell  Z0=48-Ohm
MSD_D3RFL2_60_PU500   LPDDR2 MSD_D3R_PDIFF_PDQSR cell  Z0=60-Ohm
MSD_D3RFL2_80_PU500   LPDDR2 MSD_D3R_PDIFF_PDQSR cell  Z0=80-Ohm
MSD_D3RFL_48_PU500   LPDDR MSD_D3R_PDIFF_PDQSR cell  Z0=48-Ohm
MSD_D3RFL2_34_PU550   LPDDR2 MSD_D3R_PDIFF_PDQSR cell  Z0=34-Ohm
MSD_D3RFL2_40_PU550   LPDDR2 MSD_D3R_PDIFF_PDQSR cell  Z0=40-Ohm
MSD_D3RFL2_48_PU550   LPDDR2 MSD_D3R_PDIFF_PDQSR cell  Z0=48-Ohm
MSD_D3RFL2_60_PU550   LPDDR2 MSD_D3R_PDIFF_PDQSR cell  Z0=60-Ohm
MSD_D3RFL2_80_PU550   LPDDR2 MSD_D3R_PDIFF_PDQSR cell  Z0=80-Ohm
MSD_D3RFL_48_PU550   LPDDR MSD_D3R_PDIFF_PDQSR cell  Z0=48-Ohm
MSD_D3RFL2_34_PU611   LPDDR2 MSD_D3R_PDIFF_PDQSR cell  Z0=34-Ohm
MSD_D3RFL2_40_PU611   LPDDR2 MSD_D3R_PDIFF_PDQSR cell  Z0=40-Ohm
MSD_D3RFL2_48_PU611   LPDDR2 MSD_D3R_PDIFF_PDQSR cell  Z0=48-Ohm
MSD_D3RFL2_60_PU611   LPDDR2 MSD_D3R_PDIFF_PDQSR cell  Z0=60-Ohm
MSD_D3RFL2_80_PU611   LPDDR2 MSD_D3R_PDIFF_PDQSR cell  Z0=80-Ohm
MSD_D3RFL_48_PU611   LPDDR MSD_D3R_PDIFF_PDQSR cell  Z0=48-Ohm
MSD_D3RFL2_34_PU688   LPDDR2 MSD_D3R_PDIFF_PDQSR cell  Z0=34-Ohm
MSD_D3RFL2_40_PU688   LPDDR2 MSD_D3R_PDIFF_PDQSR cell  Z0=40-Ohm
MSD_D3RFL2_48_PU688   LPDDR2 MSD_D3R_PDIFF_PDQSR cell  Z0=48-Ohm
MSD_D3RFL2_60_PU688   LPDDR2 MSD_D3R_PDIFF_PDQSR cell  Z0=60-Ohm
MSD_D3RFL2_80_PU688   LPDDR2 MSD_D3R_PDIFF_PDQSR cell  Z0=80-Ohm
MSD_D3RFL_48_PU688   LPDDR MSD_D3R_PDIFF_PDQSR cell  Z0=48-Ohm
MSD_D3RFL2_34_PWRDWN   LPDDR2 MSD_D3R_PDIFF_PDQSR cell  Z0=34-Ohm
MSD_D3RFL2_40_PWRDWN   LPDDR2 MSD_D3R_PDIFF_PDQSR cell  Z0=40-Ohm
MSD_D3RFL2_48_PWRDWN   LPDDR2 MSD_D3R_PDIFF_PDQSR cell  Z0=48-Ohm
MSD_D3RFL2_60_PWRDWN   LPDDR2 MSD_D3R_PDIFF_PDQSR cell  Z0=60-Ohm
MSD_D3RFL2_80_PWRDWN   LPDDR2 MSD_D3R_PDIFF_PDQSR cell  Z0=80-Ohm
MSD_D3RFL_48_PWRDWN   LPDDR MSD_D3R_PDIFF_PDQSR cell  Z0=48-Ohm
MSD_D3RF2_ODT150_OPEN   DDR2 MSD_D3R_PDIFF_PDQSR cell 150-Ohm ODT Receiver
MSD_D3RF2_ODT50_OPEN   DDR2 MSD_D3R_PDIFF_PDQSR cell 50-Ohm ODT Receiver
MSD_D3RF2_ODT75_OPEN   DDR2 MSD_D3R_PDIFF_PDQSR cell 75-Ohm ODT Receiver
MSD_D3RF2_ODTOFF_OPEN   DDR2 MSD_D3R_PDIFF_PDQSR cell ODT off Receiver
MSD_D3RF2_ODT150_PD344   DDR2 MSD_D3R_PDIFF_PDQSR cell 150-Ohm ODT Receiver
MSD_D3RF2_ODT50_PD344   DDR2 MSD_D3R_PDIFF_PDQSR cell 50-Ohm ODT Receiver
MSD_D3RF2_ODT75_PD344   DDR2 MSD_D3R_PDIFF_PDQSR cell 75-Ohm ODT Receiver
MSD_D3RF2_ODTOFF_PD344   DDR2 MSD_D3R_PDIFF_PDQSR cell ODT off Receiver
MSD_D3RF2_ODT150_PD393   DDR2 MSD_D3R_PDIFF_PDQSR cell 150-Ohm ODT Receiver
MSD_D3RF2_ODT50_PD393   DDR2 MSD_D3R_PDIFF_PDQSR cell 50-Ohm ODT Receiver
MSD_D3RF2_ODT75_PD393   DDR2 MSD_D3R_PDIFF_PDQSR cell 75-Ohm ODT Receiver
MSD_D3RF2_ODTOFF_PD393   DDR2 MSD_D3R_PDIFF_PDQSR cell ODT off Receiver
MSD_D3RF2_ODT150_PD458   DDR2 MSD_D3R_PDIFF_PDQSR cell 150-Ohm ODT Receiver
MSD_D3RF2_ODT50_PD458   DDR2 MSD_D3R_PDIFF_PDQSR cell 50-Ohm ODT Receiver
MSD_D3RF2_ODT75_PD458   DDR2 MSD_D3R_PDIFF_PDQSR cell 75-Ohm ODT Receiver
MSD_D3RF2_ODTOFF_PD458   DDR2 MSD_D3R_PDIFF_PDQSR cell ODT off Receiver
MSD_D3RF2_ODT150_PD500   DDR2 MSD_D3R_PDIFF_PDQSR cell 150-Ohm ODT Receiver
MSD_D3RF2_ODT50_PD500   DDR2 MSD_D3R_PDIFF_PDQSR cell 50-Ohm ODT Receiver
MSD_D3RF2_ODT75_PD500   DDR2 MSD_D3R_PDIFF_PDQSR cell 75-Ohm ODT Receiver
MSD_D3RF2_ODTOFF_PD500   DDR2 MSD_D3R_PDIFF_PDQSR cell ODT off Receiver
MSD_D3RF2_ODT150_PD550   DDR2 MSD_D3R_PDIFF_PDQSR cell 150-Ohm ODT Receiver
MSD_D3RF2_ODT50_PD550   DDR2 MSD_D3R_PDIFF_PDQSR cell 50-Ohm ODT Receiver
MSD_D3RF2_ODT75_PD550   DDR2 MSD_D3R_PDIFF_PDQSR cell 75-Ohm ODT Receiver
MSD_D3RF2_ODTOFF_PD550   DDR2 MSD_D3R_PDIFF_PDQSR cell ODT off Receiver
MSD_D3RF2_ODT150_PD611   DDR2 MSD_D3R_PDIFF_PDQSR cell 150-Ohm ODT Receiver
MSD_D3RF2_ODT50_PD611   DDR2 MSD_D3R_PDIFF_PDQSR cell 50-Ohm ODT Receiver
MSD_D3RF2_ODT75_PD611   DDR2 MSD_D3R_PDIFF_PDQSR cell 75-Ohm ODT Receiver
MSD_D3RF2_ODTOFF_PD611   DDR2 MSD_D3R_PDIFF_PDQSR cell ODT off Receiver
MSD_D3RF2_ODT150_PD688   DDR2 MSD_D3R_PDIFF_PDQSR cell 150-Ohm ODT Receiver
MSD_D3RF2_ODT50_PD688   DDR2 MSD_D3R_PDIFF_PDQSR cell 50-Ohm ODT Receiver
MSD_D3RF2_ODT75_PD688   DDR2 MSD_D3R_PDIFF_PDQSR cell 75-Ohm ODT Receiver
MSD_D3RF2_ODTOFF_PD688   DDR2 MSD_D3R_PDIFF_PDQSR cell ODT off Receiver
MSD_D3RF2_ODT150_PU344   DDR2 MSD_D3R_PDIFF_PDQSR cell 150-Ohm ODT Receiver
MSD_D3RF2_ODT50_PU344   DDR2 MSD_D3R_PDIFF_PDQSR cell 50-Ohm ODT Receiver
MSD_D3RF2_ODT75_PU344   DDR2 MSD_D3R_PDIFF_PDQSR cell 75-Ohm ODT Receiver
MSD_D3RF2_ODTOFF_PU344   DDR2 MSD_D3R_PDIFF_PDQSR cell ODT off Receiver
MSD_D3RF2_ODT150_PU393   DDR2 MSD_D3R_PDIFF_PDQSR cell 150-Ohm ODT Receiver
MSD_D3RF2_ODT50_PU393   DDR2 MSD_D3R_PDIFF_PDQSR cell 50-Ohm ODT Receiver
MSD_D3RF2_ODT75_PU393   DDR2 MSD_D3R_PDIFF_PDQSR cell 75-Ohm ODT Receiver
MSD_D3RF2_ODTOFF_PU393   DDR2 MSD_D3R_PDIFF_PDQSR cell ODT off Receiver
MSD_D3RF2_ODT150_PU458   DDR2 MSD_D3R_PDIFF_PDQSR cell 150-Ohm ODT Receiver
MSD_D3RF2_ODT50_PU458   DDR2 MSD_D3R_PDIFF_PDQSR cell 50-Ohm ODT Receiver
MSD_D3RF2_ODT75_PU458   DDR2 MSD_D3R_PDIFF_PDQSR cell 75-Ohm ODT Receiver
MSD_D3RF2_ODTOFF_PU458   DDR2 MSD_D3R_PDIFF_PDQSR cell ODT off Receiver
MSD_D3RF2_ODT150_PU500   DDR2 MSD_D3R_PDIFF_PDQSR cell 150-Ohm ODT Receiver
MSD_D3RF2_ODT50_PU500   DDR2 MSD_D3R_PDIFF_PDQSR cell 50-Ohm ODT Receiver
MSD_D3RF2_ODT75_PU500   DDR2 MSD_D3R_PDIFF_PDQSR cell 75-Ohm ODT Receiver
MSD_D3RF2_ODTOFF_PU500   DDR2 MSD_D3R_PDIFF_PDQSR cell ODT off Receiver
MSD_D3RF2_ODT150_PU550   DDR2 MSD_D3R_PDIFF_PDQSR cell 150-Ohm ODT Receiver
MSD_D3RF2_ODT50_PU550   DDR2 MSD_D3R_PDIFF_PDQSR cell 50-Ohm ODT Receiver
MSD_D3RF2_ODT75_PU550   DDR2 MSD_D3R_PDIFF_PDQSR cell 75-Ohm ODT Receiver
MSD_D3RF2_ODTOFF_PU550   DDR2 MSD_D3R_PDIFF_PDQSR cell ODT off Receiver
MSD_D3RF2_ODT150_PU611   DDR2 MSD_D3R_PDIFF_PDQSR cell 150-Ohm ODT Receiver
MSD_D3RF2_ODT50_PU611   DDR2 MSD_D3R_PDIFF_PDQSR cell 50-Ohm ODT Receiver
MSD_D3RF2_ODT75_PU611   DDR2 MSD_D3R_PDIFF_PDQSR cell 75-Ohm ODT Receiver
MSD_D3RF2_ODTOFF_PU611   DDR2 MSD_D3R_PDIFF_PDQSR cell ODT off Receiver
MSD_D3RF2_ODT150_PU688   DDR2 MSD_D3R_PDIFF_PDQSR cell 150-Ohm ODT Receiver
MSD_D3RF2_ODT50_PU688   DDR2 MSD_D3R_PDIFF_PDQSR cell 50-Ohm ODT Receiver
MSD_D3RF2_ODT75_PU688   DDR2 MSD_D3R_PDIFF_PDQSR cell 75-Ohm ODT Receiver
MSD_D3RF2_ODTOFF_PU688   DDR2 MSD_D3R_PDIFF_PDQSR cell ODT off Receiver
MSD_D3RF2_ODT150_PWRDWN   DDR2 MSD_D3R_PDIFF_PDQSR cell 150-Ohm ODT Receiver
MSD_D3RF2_ODT50_PWRDWN   DDR2 MSD_D3R_PDIFF_PDQSR cell 50-Ohm ODT Receiver
MSD_D3RF2_ODT75_PWRDWN   DDR2 MSD_D3R_PDIFF_PDQSR cell 75-Ohm ODT Receiver
MSD_D3RF2_ODTOFF_PWRDWN   DDR2 MSD_D3R_PDIFF_PDQSR cell ODT off Receiver
MSD_D3RF3_ODT120_OPEN   DDR3 MSD_D3R_PDIFF_PDQSR cell 120-Ohm ODT Receiver
MSD_D3RF3_ODT40_OPEN   DDR3 MSD_D3R_PDIFF_PDQSR cell 40-Ohm ODT Receiver
MSD_D3RF3_ODT60_OPEN   DDR3 MSD_D3R_PDIFF_PDQSR cell 60-Ohm ODT Receiver
MSD_D3RF3_ODTOFF_OPEN   DDR3 MSD_D3R_PDIFF_PDQSR cell ODT off Receiver
MSD_D3RF3_ODT120_PD344   DDR3 MSD_D3R_PDIFF_PDQSR cell 120-Ohm ODT Receiver
MSD_D3RF3_ODT40_PD344   DDR3 MSD_D3R_PDIFF_PDQSR cell 40-Ohm ODT Receiver
MSD_D3RF3_ODT60_PD344   DDR3 MSD_D3R_PDIFF_PDQSR cell 60-Ohm ODT Receiver
MSD_D3RF3_ODTOFF_PD344   DDR3 MSD_D3R_PDIFF_PDQSR cell ODT off Receiver
MSD_D3RF3_ODT120_PD393   DDR3 MSD_D3R_PDIFF_PDQSR cell 120-Ohm ODT Receiver
MSD_D3RF3_ODT40_PD393   DDR3 MSD_D3R_PDIFF_PDQSR cell 40-Ohm ODT Receiver
MSD_D3RF3_ODT60_PD393   DDR3 MSD_D3R_PDIFF_PDQSR cell 60-Ohm ODT Receiver
MSD_D3RF3_ODTOFF_PD393   DDR3 MSD_D3R_PDIFF_PDQSR cell ODT off Receiver
MSD_D3RF3_ODT120_PD458   DDR3 MSD_D3R_PDIFF_PDQSR cell 120-Ohm ODT Receiver
MSD_D3RF3_ODT40_PD458   DDR3 MSD_D3R_PDIFF_PDQSR cell 40-Ohm ODT Receiver
MSD_D3RF3_ODT60_PD458   DDR3 MSD_D3R_PDIFF_PDQSR cell 60-Ohm ODT Receiver
MSD_D3RF3_ODTOFF_PD458   DDR3 MSD_D3R_PDIFF_PDQSR cell ODT off Receiver
MSD_D3RF3_ODT120_PD500   DDR3 MSD_D3R_PDIFF_PDQSR cell 120-Ohm ODT Receiver
MSD_D3RF3_ODT40_PD500   DDR3 MSD_D3R_PDIFF_PDQSR cell 40-Ohm ODT Receiver
MSD_D3RF3_ODT60_PD500   DDR3 MSD_D3R_PDIFF_PDQSR cell 60-Ohm ODT Receiver
MSD_D3RF3_ODTOFF_PD500   DDR3 MSD_D3R_PDIFF_PDQSR cell ODT off Receiver
MSD_D3RF3_ODT120_PD550   DDR3 MSD_D3R_PDIFF_PDQSR cell 120-Ohm ODT Receiver
MSD_D3RF3_ODT40_PD550   DDR3 MSD_D3R_PDIFF_PDQSR cell 40-Ohm ODT Receiver
MSD_D3RF3_ODT60_PD550   DDR3 MSD_D3R_PDIFF_PDQSR cell 60-Ohm ODT Receiver
MSD_D3RF3_ODTOFF_PD550   DDR3 MSD_D3R_PDIFF_PDQSR cell ODT off Receiver
MSD_D3RF3_ODT120_PD611   DDR3 MSD_D3R_PDIFF_PDQSR cell 120-Ohm ODT Receiver
MSD_D3RF3_ODT40_PD611   DDR3 MSD_D3R_PDIFF_PDQSR cell 40-Ohm ODT Receiver
MSD_D3RF3_ODT60_PD611   DDR3 MSD_D3R_PDIFF_PDQSR cell 60-Ohm ODT Receiver
MSD_D3RF3_ODTOFF_PD611   DDR3 MSD_D3R_PDIFF_PDQSR cell ODT off Receiver
MSD_D3RF3_ODT120_PD688   DDR3 MSD_D3R_PDIFF_PDQSR cell 120-Ohm ODT Receiver
MSD_D3RF3_ODT40_PD688   DDR3 MSD_D3R_PDIFF_PDQSR cell 40-Ohm ODT Receiver
MSD_D3RF3_ODT60_PD688   DDR3 MSD_D3R_PDIFF_PDQSR cell 60-Ohm ODT Receiver
MSD_D3RF3_ODTOFF_PD688   DDR3 MSD_D3R_PDIFF_PDQSR cell ODT off Receiver
MSD_D3RF3_ODT120_PU344   DDR3 MSD_D3R_PDIFF_PDQSR cell 120-Ohm ODT Receiver
MSD_D3RF3_ODT40_PU344   DDR3 MSD_D3R_PDIFF_PDQSR cell 40-Ohm ODT Receiver
MSD_D3RF3_ODT60_PU344   DDR3 MSD_D3R_PDIFF_PDQSR cell 60-Ohm ODT Receiver
MSD_D3RF3_ODTOFF_PU344   DDR3 MSD_D3R_PDIFF_PDQSR cell ODT off Receiver
MSD_D3RF3_ODT120_PU393   DDR3 MSD_D3R_PDIFF_PDQSR cell 120-Ohm ODT Receiver
MSD_D3RF3_ODT40_PU393   DDR3 MSD_D3R_PDIFF_PDQSR cell 40-Ohm ODT Receiver
MSD_D3RF3_ODT60_PU393   DDR3 MSD_D3R_PDIFF_PDQSR cell 60-Ohm ODT Receiver
MSD_D3RF3_ODTOFF_PU393   DDR3 MSD_D3R_PDIFF_PDQSR cell ODT off Receiver
MSD_D3RF3_ODT120_PU458   DDR3 MSD_D3R_PDIFF_PDQSR cell 120-Ohm ODT Receiver
MSD_D3RF3_ODT40_PU458   DDR3 MSD_D3R_PDIFF_PDQSR cell 40-Ohm ODT Receiver
MSD_D3RF3_ODT60_PU458   DDR3 MSD_D3R_PDIFF_PDQSR cell 60-Ohm ODT Receiver
MSD_D3RF3_ODTOFF_PU458   DDR3 MSD_D3R_PDIFF_PDQSR cell ODT off Receiver
MSD_D3RF3_ODT120_PU500   DDR3 MSD_D3R_PDIFF_PDQSR cell 120-Ohm ODT Receiver
MSD_D3RF3_ODT40_PU500   DDR3 MSD_D3R_PDIFF_PDQSR cell 40-Ohm ODT Receiver
MSD_D3RF3_ODT60_PU500   DDR3 MSD_D3R_PDIFF_PDQSR cell 60-Ohm ODT Receiver
MSD_D3RF3_ODTOFF_PU500   DDR3 MSD_D3R_PDIFF_PDQSR cell ODT off Receiver
MSD_D3RF3_ODT120_PU550   DDR3 MSD_D3R_PDIFF_PDQSR cell 120-Ohm ODT Receiver
MSD_D3RF3_ODT40_PU550   DDR3 MSD_D3R_PDIFF_PDQSR cell 40-Ohm ODT Receiver
MSD_D3RF3_ODT60_PU550   DDR3 MSD_D3R_PDIFF_PDQSR cell 60-Ohm ODT Receiver
MSD_D3RF3_ODTOFF_PU550   DDR3 MSD_D3R_PDIFF_PDQSR cell ODT off Receiver
MSD_D3RF3_ODT120_PU611   DDR3 MSD_D3R_PDIFF_PDQSR cell 120-Ohm ODT Receiver
MSD_D3RF3_ODT40_PU611   DDR3 MSD_D3R_PDIFF_PDQSR cell 40-Ohm ODT Receiver
MSD_D3RF3_ODT60_PU611   DDR3 MSD_D3R_PDIFF_PDQSR cell 60-Ohm ODT Receiver
MSD_D3RF3_ODTOFF_PU611   DDR3 MSD_D3R_PDIFF_PDQSR cell ODT off Receiver
MSD_D3RF3_ODT120_PU688   DDR3 MSD_D3R_PDIFF_PDQSR cell 120-Ohm ODT Receiver
MSD_D3RF3_ODT40_PU688   DDR3 MSD_D3R_PDIFF_PDQSR cell 40-Ohm ODT Receiver
MSD_D3RF3_ODT60_PU688   DDR3 MSD_D3R_PDIFF_PDQSR cell 60-Ohm ODT Receiver
MSD_D3RF3_ODTOFF_PU688   DDR3 MSD_D3R_PDIFF_PDQSR cell ODT off Receiver
MSD_D3RF3_ODT120_PWRDWN   DDR3 MSD_D3R_PDIFF_PDQSR cell 120-Ohm ODT Receiver
MSD_D3RF3_ODT40_PWRDWN   DDR3 MSD_D3R_PDIFF_PDQSR cell 40-Ohm ODT Receiver
MSD_D3RF3_ODT60_PWRDWN   DDR3 MSD_D3R_PDIFF_PDQSR cell 60-Ohm ODT Receiver
MSD_D3RF3_ODTOFF_PWRDWN   DDR3 MSD_D3R_PDIFF_PDQSR cell ODT off Receiver
MSD_D3RF3L_ODT120_OPEN   DDR3L MSD_D3R_PDIFF_PDQSR cell 120-Ohm ODT Receiver
MSD_D3RF3L_ODT40_OPEN   DDR3L MSD_D3R_PDIFF_PDQSR cell 40-Ohm ODT Receiver
MSD_D3RF3L_ODT60_OPEN   DDR3L MSD_D3R_PDIFF_PDQSR cell 60-Ohm ODT Receiver
MSD_D3RF3L_ODTOFF_OPEN   DDR3L MSD_D3R_PDIFF_PDQSR cell ODT off Receiver
MSD_D3RF3L_ODT120_PD344   DDR3L MSD_D3R_PDIFF_PDQSR cell 120-Ohm ODT Receiver
MSD_D3RF3L_ODT40_PD344   DDR3L MSD_D3R_PDIFF_PDQSR cell 40-Ohm ODT Receiver
MSD_D3RF3L_ODT60_PD344   DDR3L MSD_D3R_PDIFF_PDQSR cell 60-Ohm ODT Receiver
MSD_D3RF3L_ODTOFF_PD344   DDR3L MSD_D3R_PDIFF_PDQSR cell ODT off Receiver
MSD_D3RF3L_ODT120_PD393   DDR3L MSD_D3R_PDIFF_PDQSR cell 120-Ohm ODT Receiver
MSD_D3RF3L_ODT40_PD393   DDR3L MSD_D3R_PDIFF_PDQSR cell 40-Ohm ODT Receiver
MSD_D3RF3L_ODT60_PD393   DDR3L MSD_D3R_PDIFF_PDQSR cell 60-Ohm ODT Receiver
MSD_D3RF3L_ODTOFF_PD393   DDR3L MSD_D3R_PDIFF_PDQSR cell ODT off Receiver
MSD_D3RF3L_ODT120_PD458   DDR3L MSD_D3R_PDIFF_PDQSR cell 120-Ohm ODT Receiver
MSD_D3RF3L_ODT40_PD458   DDR3L MSD_D3R_PDIFF_PDQSR cell 40-Ohm ODT Receiver
MSD_D3RF3L_ODT60_PD458   DDR3L MSD_D3R_PDIFF_PDQSR cell 60-Ohm ODT Receiver
MSD_D3RF3L_ODTOFF_PD458   DDR3L MSD_D3R_PDIFF_PDQSR cell ODT off Receiver
MSD_D3RF3L_ODT120_PD500   DDR3L MSD_D3R_PDIFF_PDQSR cell 120-Ohm ODT Receiver
MSD_D3RF3L_ODT40_PD500   DDR3L MSD_D3R_PDIFF_PDQSR cell 40-Ohm ODT Receiver
MSD_D3RF3L_ODT60_PD500   DDR3L MSD_D3R_PDIFF_PDQSR cell 60-Ohm ODT Receiver
MSD_D3RF3L_ODTOFF_PD500   DDR3L MSD_D3R_PDIFF_PDQSR cell ODT off Receiver
MSD_D3RF3L_ODT120_PD550   DDR3L MSD_D3R_PDIFF_PDQSR cell 120-Ohm ODT Receiver
MSD_D3RF3L_ODT40_PD550   DDR3L MSD_D3R_PDIFF_PDQSR cell 40-Ohm ODT Receiver
MSD_D3RF3L_ODT60_PD550   DDR3L MSD_D3R_PDIFF_PDQSR cell 60-Ohm ODT Receiver
MSD_D3RF3L_ODTOFF_PD550   DDR3L MSD_D3R_PDIFF_PDQSR cell ODT off Receiver
MSD_D3RF3L_ODT120_PD611   DDR3L MSD_D3R_PDIFF_PDQSR cell 120-Ohm ODT Receiver
MSD_D3RF3L_ODT40_PD611   DDR3L MSD_D3R_PDIFF_PDQSR cell 40-Ohm ODT Receiver
MSD_D3RF3L_ODT60_PD611   DDR3L MSD_D3R_PDIFF_PDQSR cell 60-Ohm ODT Receiver
MSD_D3RF3L_ODTOFF_PD611   DDR3L MSD_D3R_PDIFF_PDQSR cell ODT off Receiver
MSD_D3RF3L_ODT120_PD688   DDR3L MSD_D3R_PDIFF_PDQSR cell 120-Ohm ODT Receiver
MSD_D3RF3L_ODT40_PD688   DDR3L MSD_D3R_PDIFF_PDQSR cell 40-Ohm ODT Receiver
MSD_D3RF3L_ODT60_PD688   DDR3L MSD_D3R_PDIFF_PDQSR cell 60-Ohm ODT Receiver
MSD_D3RF3L_ODTOFF_PD688   DDR3L MSD_D3R_PDIFF_PDQSR cell ODT off Receiver
MSD_D3RF3L_ODT120_PU344   DDR3L MSD_D3R_PDIFF_PDQSR cell 120-Ohm ODT Receiver
MSD_D3RF3L_ODT40_PU344   DDR3L MSD_D3R_PDIFF_PDQSR cell 40-Ohm ODT Receiver
MSD_D3RF3L_ODT60_PU344   DDR3L MSD_D3R_PDIFF_PDQSR cell 60-Ohm ODT Receiver
MSD_D3RF3L_ODTOFF_PU344   DDR3L MSD_D3R_PDIFF_PDQSR cell ODT off Receiver
MSD_D3RF3L_ODT120_PU393   DDR3L MSD_D3R_PDIFF_PDQSR cell 120-Ohm ODT Receiver
MSD_D3RF3L_ODT40_PU393   DDR3L MSD_D3R_PDIFF_PDQSR cell 40-Ohm ODT Receiver
MSD_D3RF3L_ODT60_PU393   DDR3L MSD_D3R_PDIFF_PDQSR cell 60-Ohm ODT Receiver
MSD_D3RF3L_ODTOFF_PU393   DDR3L MSD_D3R_PDIFF_PDQSR cell ODT off Receiver
MSD_D3RF3L_ODT120_PU458   DDR3L MSD_D3R_PDIFF_PDQSR cell 120-Ohm ODT Receiver
MSD_D3RF3L_ODT40_PU458   DDR3L MSD_D3R_PDIFF_PDQSR cell 40-Ohm ODT Receiver
MSD_D3RF3L_ODT60_PU458   DDR3L MSD_D3R_PDIFF_PDQSR cell 60-Ohm ODT Receiver
MSD_D3RF3L_ODTOFF_PU458   DDR3L MSD_D3R_PDIFF_PDQSR cell ODT off Receiver
MSD_D3RF3L_ODT120_PU500   DDR3L MSD_D3R_PDIFF_PDQSR cell 120-Ohm ODT Receiver
MSD_D3RF3L_ODT40_PU500   DDR3L MSD_D3R_PDIFF_PDQSR cell 40-Ohm ODT Receiver
MSD_D3RF3L_ODT60_PU500   DDR3L MSD_D3R_PDIFF_PDQSR cell 60-Ohm ODT Receiver
MSD_D3RF3L_ODTOFF_PU500   DDR3L MSD_D3R_PDIFF_PDQSR cell ODT off Receiver
MSD_D3RF3L_ODT120_PU550   DDR3L MSD_D3R_PDIFF_PDQSR cell 120-Ohm ODT Receiver
MSD_D3RF3L_ODT40_PU550   DDR3L MSD_D3R_PDIFF_PDQSR cell 40-Ohm ODT Receiver
MSD_D3RF3L_ODT60_PU550   DDR3L MSD_D3R_PDIFF_PDQSR cell 60-Ohm ODT Receiver
MSD_D3RF3L_ODTOFF_PU550   DDR3L MSD_D3R_PDIFF_PDQSR cell ODT off Receiver
MSD_D3RF3L_ODT120_PU611   DDR3L MSD_D3R_PDIFF_PDQSR cell 120-Ohm ODT Receiver
MSD_D3RF3L_ODT40_PU611   DDR3L MSD_D3R_PDIFF_PDQSR cell 40-Ohm ODT Receiver
MSD_D3RF3L_ODT60_PU611   DDR3L MSD_D3R_PDIFF_PDQSR cell 60-Ohm ODT Receiver
MSD_D3RF3L_ODTOFF_PU611   DDR3L MSD_D3R_PDIFF_PDQSR cell ODT off Receiver
MSD_D3RF3L_ODT120_PU688   DDR3L MSD_D3R_PDIFF_PDQSR cell 120-Ohm ODT Receiver
MSD_D3RF3L_ODT40_PU688   DDR3L MSD_D3R_PDIFF_PDQSR cell 40-Ohm ODT Receiver
MSD_D3RF3L_ODT60_PU688   DDR3L MSD_D3R_PDIFF_PDQSR cell 60-Ohm ODT Receiver
MSD_D3RF3L_ODTOFF_PU688   DDR3L MSD_D3R_PDIFF_PDQSR cell ODT off Receiver
MSD_D3RF3L_ODT120_PWRDWN   DDR3L MSD_D3R_PDIFF_PDQSR cell 120-Ohm ODT Receiver
MSD_D3RF3L_ODT40_PWRDWN   DDR3L MSD_D3R_PDIFF_PDQSR cell 40-Ohm ODT Receiver
MSD_D3RF3L_ODT60_PWRDWN   DDR3L MSD_D3R_PDIFF_PDQSR cell 60-Ohm ODT Receiver
MSD_D3RF3L_ODTOFF_PWRDWN   DDR3L MSD_D3R_PDIFF_PDQSR cell ODT off Receiver
MSD_D3RFL2_ODTOFF_OPEN   LPDDR2 MSD_D3R_PDIFF_PDQSR cell ODT off Receiver
MSD_D3RFL_ODTOFF_OPEN   LPDDR MSD_D3R_PDIFF_PDQSR cell ODT off Receiver
MSD_D3RFL2_ODTOFF_PD344   LPDDR2 MSD_D3R_PDIFF_PDQSR cell ODT off Receiver
MSD_D3RFL_ODTOFF_PD344   LPDDR MSD_D3R_PDIFF_PDQSR cell ODT off Receiver
MSD_D3RFL2_ODTOFF_PD393   LPDDR2 MSD_D3R_PDIFF_PDQSR cell ODT off Receiver
MSD_D3RFL_ODTOFF_PD393   LPDDR MSD_D3R_PDIFF_PDQSR cell ODT off Receiver
MSD_D3RFL2_ODTOFF_PD458   LPDDR2 MSD_D3R_PDIFF_PDQSR cell ODT off Receiver
MSD_D3RFL_ODTOFF_PD458   LPDDR MSD_D3R_PDIFF_PDQSR cell ODT off Receiver
MSD_D3RFL2_ODTOFF_PD500   LPDDR2 MSD_D3R_PDIFF_PDQSR cell ODT off Receiver
MSD_D3RFL_ODTOFF_PD500   LPDDR MSD_D3R_PDIFF_PDQSR cell ODT off Receiver
MSD_D3RFL2_ODTOFF_PD550   LPDDR2 MSD_D3R_PDIFF_PDQSR cell ODT off Receiver
MSD_D3RFL_ODTOFF_PD550   LPDDR MSD_D3R_PDIFF_PDQSR cell ODT off Receiver
MSD_D3RFL2_ODTOFF_PD611   LPDDR2 MSD_D3R_PDIFF_PDQSR cell ODT off Receiver
MSD_D3RFL_ODTOFF_PD611   LPDDR MSD_D3R_PDIFF_PDQSR cell ODT off Receiver
MSD_D3RFL2_ODTOFF_PD688   LPDDR2 MSD_D3R_PDIFF_PDQSR cell ODT off Receiver
MSD_D3RFL_ODTOFF_PD688   LPDDR MSD_D3R_PDIFF_PDQSR cell ODT off Receiver
MSD_D3RFL2_ODTOFF_PU344   LPDDR2 MSD_D3R_PDIFF_PDQSR cell ODT off Receiver
MSD_D3RFL_ODTOFF_PU344   LPDDR MSD_D3R_PDIFF_PDQSR cell ODT off Receiver
MSD_D3RFL2_ODTOFF_PU393   LPDDR2 MSD_D3R_PDIFF_PDQSR cell ODT off Receiver
MSD_D3RFL_ODTOFF_PU393   LPDDR MSD_D3R_PDIFF_PDQSR cell ODT off Receiver
MSD_D3RFL2_ODTOFF_PU458   LPDDR2 MSD_D3R_PDIFF_PDQSR cell ODT off Receiver
MSD_D3RFL_ODTOFF_PU458   LPDDR MSD_D3R_PDIFF_PDQSR cell ODT off Receiver
MSD_D3RFL2_ODTOFF_PU500   LPDDR2 MSD_D3R_PDIFF_PDQSR cell ODT off Receiver
MSD_D3RFL_ODTOFF_PU500   LPDDR MSD_D3R_PDIFF_PDQSR cell ODT off Receiver
MSD_D3RFL2_ODTOFF_PU550   LPDDR2 MSD_D3R_PDIFF_PDQSR cell ODT off Receiver
MSD_D3RFL_ODTOFF_PU550   LPDDR MSD_D3R_PDIFF_PDQSR cell ODT off Receiver
MSD_D3RFL2_ODTOFF_PU611   LPDDR2 MSD_D3R_PDIFF_PDQSR cell ODT off Receiver
MSD_D3RFL_ODTOFF_PU611   LPDDR MSD_D3R_PDIFF_PDQSR cell ODT off Receiver
MSD_D3RFL2_ODTOFF_PU688   LPDDR2 MSD_D3R_PDIFF_PDQSR cell ODT off Receiver
MSD_D3RFL_ODTOFF_PU688   LPDDR MSD_D3R_PDIFF_PDQSR cell ODT off Receiver
MSD_D3RFL2_ODTOFF_PWRDWN   LPDDR2 MSD_D3R_PDIFF_PDQSR cell ODT off Receiver
MSD_D3RFL_ODTOFF_PWRDWN   LPDDR MSD_D3R_PDIFF_PDQSR cell ODT off Receiver
[Model Selector] PDDRIO_PAD
MSD_D3RP2_18   DDR2 MSD_D3R_PDDRIO Z0=18-Ohm
MSD_D3RP2_40   DDR2 MSD_D3R_PDDRIO Z0=40-Ohm
MSD_D3RP2_48   DDR2 MSD_D3R_PDDRIO Z0=48-Ohm
MSD_D3RP2_ODT150   DDR2 MSD_D3R_PDDRIO cell 150-Ohm ODT Receiver
MSD_D3RP2_ODT50   DDR2 MSD_D3R_PDDRIO cell 50-Ohm ODT Receiver
MSD_D3RP2_ODT75   DDR2 MSD_D3R_PDDRIO cell 75-Ohm ODT Receiver
MSD_D3RP2_ODTOFF   DDR2 MSD_D3R_PDDRIO cell ODT off Receiver
MSD_D3RP3_34   DDR3 MSD_D3R_PDDRIO cell  Z0=34-Ohm
MSD_D3RP3_40   DDR3 MSD_D3R_PDDRIO cell  Z0=40-Ohm
MSD_D3RP3_48   DDR3 MSD_D3R_PDDRIO cell  Z0=48-Ohm
MSD_D3RP3L_34   DDR3L MSD_D3R_PDDRIO cell  Z0=34-Ohm
MSD_D3RP3L_40   DDR3L MSD_D3R_PDDRIO cell  Z0=40-Ohm
MSD_D3RP3L_48   DDR3L MSD_D3R_PDDRIO cell  Z0=48-Ohm
MSD_D3RP3L_ODT120   DDR3L MSD_D3R_PDDRIO cell 120-Ohm ODT Receiver
MSD_D3RP3L_ODT40   DDR3L MSD_D3R_PDDRIO cell 40-Ohm ODT Receiver
MSD_D3RP3L_ODT60   DDR3L MSD_D3R_PDDRIO cell 60-Ohm ODT Receiver
MSD_D3RP3L_ODTOFF   DDR3L MSD_D3R_PDDRIO cell ODT off Receiver
MSD_D3RP3_ODT120   DDR3 MSD_D3R_PDDRIO cell 120-Ohm ODT Receiver
MSD_D3RP3_ODT40   DDR3 MSD_D3R_PDDRIO cell 40-Ohm ODT Receiver
MSD_D3RP3_ODT60   DDR3 MSD_D3R_PDDRIO cell 60-Ohm ODT Receiver
MSD_D3RP3_ODTOFF   DDR3 MSD_D3R_PDDRIO cell ODT off Receiver
MSD_D3RPL2_34   LPDDR2 MSD_D3R_PDDRIO cell  Z0=34-Ohm
MSD_D3RPL2_40   LPDDR2 MSD_D3R_PDDRIO cell  Z0=40-Ohm
MSD_D3RPL2_48   LPDDR2 MSD_D3R_PDDRIO cell  Z0=48-Ohm
MSD_D3RPL2_60   LPDDR2 MSD_D3R_PDDRIO cell  Z0=60-Ohm
MSD_D3RPL2_80   LPDDR2 MSD_D3R_PDDRIO cell  Z0=80-Ohm
MSD_D3RPL2_ODTOFF   LPDDR2 MSD_D3R_PDDRIO cell ODT off Receiver
MSD_D3RPL_48   LPDDR MSD_D3R_PDDRIO cell  Z0=48-Ohm
MSD_D3RPL_ODTOFF   LPDDR MSD_D3R_PDDRIO cell ODT off Receiver
[Model Selector] io8_ft
io8_ft_ls_1v2   "GPIO - 5V tolerant - 1.2V range - Low speed"
io8_ft_ms_1v2   "GPIO - 5V tolerant - 1.2V range - Med speed"
io8_ft_hs_1v2   "GPIO - 5V tolerant - 1.2V range - High speed"
io8_ft_fs_1v2   "GPIO - 5V tolerant - 1.2V range - Fast speed"
io8_ft_hs_1v8   "GPIO - 5V tolerant - 1.8V range - High speed -"
io8_ft_fs_1v8   "GPIO - 5V tolerant - 1.8V range - Fast speed -"
io8_ft_ms_1v8   "GPIO - 5V tolerant - 1.8V range - Medium speed"
io8_ft_ls_1v8   "GPIO - 5V tolerant - 1.8V range - Low speed"
io8_ft_hs_3v3   "GPIO - 5V tolerant - 3.3V range - High speed"
io8_ft_fs_3v3   "GPIO - 5V tolerant - 3.3V range - Fast speed"
io8_ft_ms_3v3   "GPIO - 5V tolerant - 3.3V range - Medium speed"
io8_ft_ls_3v3   "GPIO - 5V tolerant - 3.3V range - Low speed"
[Model Selector] io8_ft_hslv
io8_ft_ls_1v2   "GPIO - 5V tolerant - 1.2V range - Low speed"
io8_ft_ms_1v2   "GPIO - 5V tolerant - 1.2V range - Med speed"
io8_ft_hs_1v2   "GPIO - 5V tolerant - 1.2V range - High speed"
io8_ft_fs_1v2   "GPIO - 5V tolerant - 1.2V range - Fast speed"
io8_ft_hs_1v8   "GPIO - 5V tolerant - 1.8V range - High speed -"
io8_ft_fs_1v8   "GPIO - 5V tolerant - 1.8V range - Fast speed -"
io8_ft_ms_1v8   "GPIO - 5V tolerant - 1.8V range - Medium speed"
io8_ft_ls_1v8   "GPIO - 5V tolerant - 1.8V range - Low speed"
io8_ft_hs_3v3   "GPIO - 5V tolerant - 3.3V range - High speed"
io8_ft_fs_3v3   "GPIO - 5V tolerant - 3.3V range - Fast speed"
io8_ft_ms_3v3   "GPIO - 5V tolerant - 3.3V range - Medium speed"
io8_ft_ls_3v3   "GPIO - 5V tolerant - 3.3V range - Low speed"
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| Models and submodels in the file (574): io8_ft_ls_1v2 (I/O), io8_ft_ms_1v2 (I/O), io8_ft_fs_1v2 (I/O), io8_ft_hs_1v2 (I/O), io8_ft_ls_1v8 (I/O), io8_ft_ms_1v8 (I/O), io8_ft_fs_1v8 (I/O), io8_ft_hs_1v8 (I/O), io8_ft_ls_3v3 (I/O), io8_ft_ms_3v3 (I/O), io8_ft_fs_3v3 (I/O), io8_ft_hs_3v3 (I/O), io8_ft_hslv_et_ls_1v2 (I/O), io8_ft_hslv_et_ms_1v2 (I/O), io8_ft_hslv_et_fs_1v2 (I/O), io8_ft_hslv_et_hs_1v2 (I/O), io8_ft_hslv_et_ls_1v8 (I/O), io8_ft_hslv_et_ms_1v8 (I/O), io8_ft_hslv_et_fs_1v8 (I/O), io8_ft_hslv_et_hs_1v8 (I/O), io8_ft_hslv_et_ls_2v5 (I/O), io8_ft_hslv_et_ms_2v5 (I/O), io8_ft_hslv_et_fs_2v5 (I/O), io8_ft_hslv_et_hs_2v5 (I/O), io8_ft_hslv_ls_1v2 (I/O), io8_ft_hslv_ms_1v2 (I/O), io8_ft_hslv_fs_1v2 (I/O), io8_ft_hslv_hs_1v2 (I/O), io8_ft_hslv_ls_1v8 (I/O), io8_ft_hslv_ms_1v8 (I/O), io8_ft_hslv_fs_1v8 (I/O), io8_ft_hslv_hs_1v8 (I/O), io8_ft_hslv_ls_2v5 (I/O), io8_ft_hslv_ms_2v5 (I/O), io8_ft_hslv_fs_2v5 (I/O), io8_ft_hslv_hs_2v5 (I/O), io8_ft_i2c_ls_1v2 (I/O_open_drain), io8_ft_i2c_ms_1v2 (I/O_open_drain), io8_ft_i2c_fs_1v2 (I/O_open_drain), io8_ft_i2c_hs_1v2 (I/O_open_drain), io8_ft_i2c_ls_1v8 (I/O_open_drain), io8_ft_i2c_ms_1v8 (I/O_open_drain), io8_ft_i2c_fs_1v8 (I/O_open_drain), io8_ft_i2c_hs_1v8 (I/O_open_drain), io8_ft_i2c_ls_3v3 (I/O_open_drain), io8_ft_i2c_ms_3v3 (I/O_open_drain), io8_ft_i2c_fs_3v3 (I/O_open_drain), io8_ft_i2c_hs_3v3 (I/O_open_drain), io8usb_adp_3v3 (I/O), io8usb_vbus_3v3 (I/O), io8usb_id_ft_nopup (Input), io8usb_id_ft_pup (Input), MSD_D3RF2_18 (I/O), MSD_D3RF2_40 (I/O), MSD_D3RF2_48 (I/O), MSD_D3RF2_ODT150 (Input), MSD_D3RF2_ODT50 (Input), MSD_D3RF2_ODT75 (Input), MSD_D3RF2_ODTOFF (Input), MSD_D3RF3_34 (I/O), MSD_D3RF3_40 (I/O), MSD_D3RF3_48 (I/O), MSD_D3RF3L_34 (I/O), MSD_D3RF3L_40 (I/O), MSD_D3RF3L_48 (I/O), MSD_D3RF3L_ODT120 (Input), MSD_D3RF3L_ODT40 (Input), MSD_D3RF3L_ODT60 (Input), MSD_D3RF3L_ODTOFF (Input), MSD_D3RF3_ODT120 (Input), MSD_D3RF3_ODT40 (Input), MSD_D3RF3_ODT60 (Input), MSD_D3RF3_ODTOFF (Input), MSD_D3RFL2_34 (I/O), MSD_D3RFL2_40 (I/O), MSD_D3RFL2_48 (I/O), MSD_D3RFL2_60 (I/O), MSD_D3RFL2_80 (I/O), MSD_D3RFL2_ODTOFF (Input), MSD_D3RFL_48 (I/O)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
